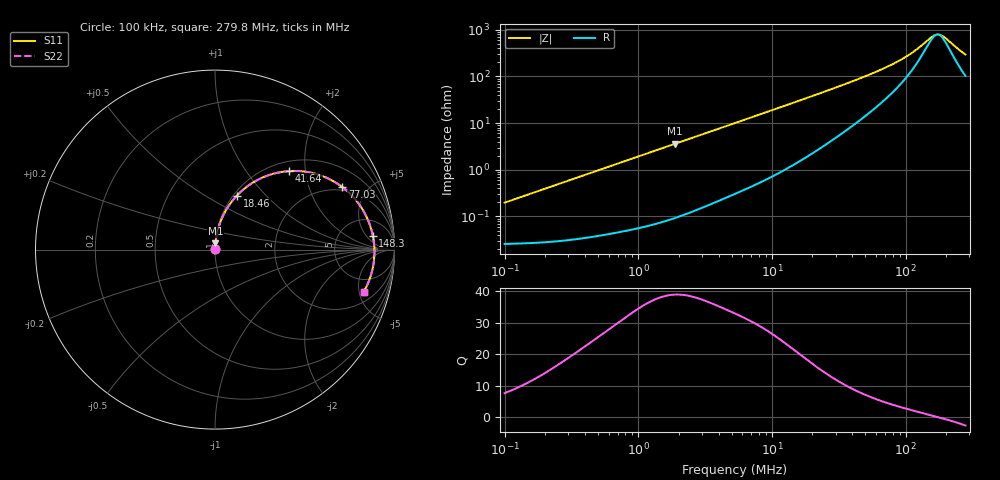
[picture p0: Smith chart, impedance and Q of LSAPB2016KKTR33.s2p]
! LSAPB2016KKTR33  S-PARAMETER MODEL  ( General Type )
! Model Generated by TAIYO YUDEN Corporation (http://www.ty-top.com)
! Version 2.0
! TAIYO YUDEN Control No. 20210629
! Copyright(c) 2015 TAIYO YUDEN CO.,LTD. All Rights Reserved.
! Product Description (link to TY-COMPAS)
! https://ds.yuden.co.jp/TYCOMPAS/or/detail?pn=LSAPB2016KKTR33M&u=M
! Products Name : Inductors
! Characteristics :
!  Inductance : 0.33 uH , SRF(min) : -Hz , DC Resistance(max) : 0.03 Ohm
!  Rated Current : Saturation :4700 mA , Temp Rise : 3500 mA (40 degC)
!  Case Size : 2.0 x 1.6 / 0.079 x 0.063 [mm/inch] , Thickness : 1 / 0.039 [mm/inch]
!  (Conditions: Temperature = 25 degC , DC Bias Current/Voltage = 0A / 0V)
! External Node Assignments :
!  1  o---GGG---o  2
! GND o---------o GND
! Frequency Range : 0.1MHz  -  279.750408MHz  [ 402 STEP ]
# MHz S RI R 50
! Freq[MHz].  S11 Real  S11 Imag  S21 Real  S21 Imag  S12 Real  S12 Imag  S22 Real  S22 Imag
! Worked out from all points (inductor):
!   401 points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, 100 kHz to 279.8 MHz, reference 50 ohm
!   read as one part in series: L = 312 nH near 104 kHz
!   highest Q = 39 at 1.885 MHz (marker M1), where L = 305 nH
!   self-resonance near 173.1 MHz
!   S11 on the Smith chart (normalised r, x): 100 kHz: 1.00, +0.00; 18.46 MHz: 1.04, +0.70; 41.64 MHz: 1.19, +1.64; 77.03 MHz: 1.82, +3.39; 148.3 MHz: 11, +7; 279.8 MHz: 3.06, -5.56
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0.1  0.000262 0.00196  0.9997 -0.00196  0.9997 -0.00196  0.000262 0.00196
0.377863  0.000392 0.00736  0.9996 -0.00736  0.9996 -0.00736  0.000392 0.00736
1.427803  0.00147 0.0274  0.9985 -0.0274  0.9985 -0.0274  0.00147 0.0274
1.884973  0.00223 0.0361  0.9978 -0.0361  0.9978 -0.0361  0.00223 0.0361
5.289144  0.0129 0.0988  0.9871 -0.0988  0.9871 -0.0988  0.0129 0.0988
11.02076  0.0487 0.1964  0.9513 -0.1964  0.9513 -0.1964  0.0487 0.1964
18.46085  0.1224 0.3012  0.8776 -0.3012  0.8776 -0.3012  0.1224 0.3012
19.9857  0.1402 0.3189  0.8598 -0.3189  0.8598 -0.3189  0.1402 0.3189
28.56434  0.2488 0.394  0.7512 -0.394  0.7512 -0.394  0.2488 0.394
41.64336  0.4137 0.4376  0.5863 -0.4376  0.5863 -0.4376  0.4137 0.4376
56.07892  0.5629 0.4216  0.4371 -0.4216  0.4371 -0.4216  0.5629 0.4216
75.51853  0.7014 0.3543  0.2986 -0.3543  0.2986 -0.3543  0.7014 0.3543
77.03188  0.7097 0.3482  0.2903 -0.3482  0.2903 -0.3482  0.7097 0.3482
92.0922  0.7765 0.2858  0.2235 -0.2858  0.2235 -0.2858  0.7765 0.2858
107.934  0.8235 0.2213  0.1765 -0.2213  0.1765 -0.2213  0.8235 0.2213
124.0157  0.8544 0.1597  0.1456 -0.1597  0.1456 -0.1597  0.8544 0.1597
148.2617  0.8796 0.0757  0.1204 -0.0757  0.1204 -0.0757  0.8796 0.0757
167.0054  0.8873 0.0177  0.1127 -0.0177  0.1127 -0.0177  0.8873 0.0177
184.4231  0.8879 -0.0313  0.1121 0.0313  0.1121 0.0313  0.8879 -0.0313
199.6563  0.8844 -0.0708  0.1156 0.0708  0.1156 0.0708  0.8844 -0.0708
253.3297  0.8522 -0.188  0.1478 0.188  0.1478 0.188  0.8522 -0.188
279.7504  0.8287 -0.2347  0.1713 0.2347  0.1713 0.2347  0.8287 -0.2347
